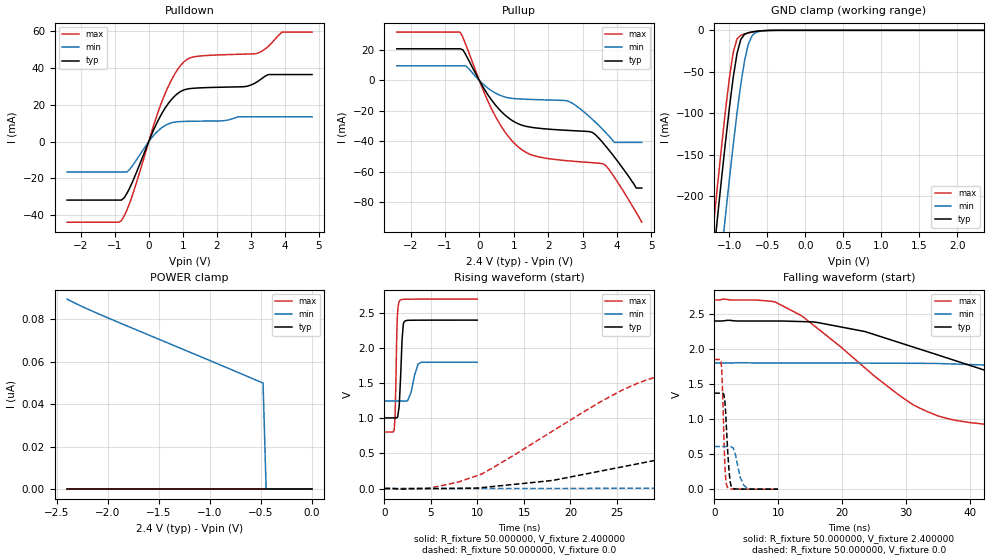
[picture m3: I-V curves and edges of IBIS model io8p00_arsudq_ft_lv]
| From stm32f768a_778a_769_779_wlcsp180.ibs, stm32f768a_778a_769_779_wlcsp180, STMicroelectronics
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|   Model io8p00_arsudq_ft_lv
[Model]  io8p00_arsudq_ft_lv
Model_type I/O
Polarity   Non-Inverting
Enable   Active-Low
Vinl =   0.720000V
Vinh =   1.680000V
Vmeas =  1.200000V
Cref =   50.000000pF
Rref =   100.000000M
Vref =   0.0V
C_comp   2.238800pF   2.178700pF   2.334000pF
[Temperature Range]   25.000000   0.125000k   -40.000000
[Pullup Reference]   2.400000V   1.800000V   2.700000V
[Pulldown Reference]   0.0V   0.0V   0.0V
[POWER Clamp Reference]   2.400000V   1.800000V   2.700000V
[GND Clamp Reference]   0.0V   0.0V   0.0V
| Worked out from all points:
|   slope of the pulldown table from 0 to 0.36 V, typ, clamps not added: 25 ohm
|   slope of the pullup table from 0 to 0.36 V, typ, clamps not added: 27.7 ohm
|   GND clamp passes 1 mA (typ) near -0.62 V on its own axis
|   rising waveform, R_fixture 50.000000, V_fixture 2.400000: 20-80 % time 271ps typ, 604ps min, 183ps max; typ from 1.01 V to 2.4 V
|   rising waveform, R_fixture 50.000000, V_fixture 0.0: 20-80 % time 32.8ns typ, 82.1ns min, 14.3ns max; typ from 0 V to 1.37 V
|   falling waveform, R_fixture 50.000000, V_fixture 2.400000: 20-80 % time 29.4ns typ, 74.3ns min, 15.7ns max; typ from 2.4 V to 1.01 V
|   falling waveform, R_fixture 50.000000, V_fixture 0.0: 20-80 % time 523ps typ, 976ps min, 385ps max; typ from 1.37 V to 0 V
[Pulldown]
|Voltage   I(typ)   I(min)   I(max)
-2.4V     -31.73mA   -16.51mA   -43.74mA
-800mV    -31.73mA   -16.51mA   -42.87mA
-480mV    -21.98mA   -13.17mA   -29.21mA
80mV      3.63mA     1.966mA    5.014mA
480mV     18.16mA    8.738mA    26.02mA
800mV     25.38mA    10.72mA    37.77mA
1.12V     28.53mA    11.02mA    44.6mA
2.8V      29.84mA    13.49mA    47.53mA
3.2V      32.65mA    13.49mA    48.05mA
3.52V     36.43mA    13.49mA    51.84mA
3.92V     36.43mA    13.49mA    59.49mA
4.8V      36.43mA    13.49mA    59.49mA
[Pullup]
|Voltage   I(typ)   I(min)   I(max)
-2.4V     20.89mA    9.66mA     31.9mA
-560mV    20.89mA    9.66mA     31.9mA
-400mV    17.28mA    9.66mA     24.07mA
320mV     -11.75mA   -6.207mA   -17.08mA
960mV     -26.47mA   -11.82mA   -40.02mA
1.52V     -30.88mA   -12.51mA   -49.05mA
2.56V     -32.88mA   -13.48mA   -52.9mA
3.28V     -34.19mA   -25.52mA   -54.18mA
3.6V      -41.31mA   -32.62mA   -54.97mA
3.92V     -50.33mA   -40.8mA    -63.62mA
4.56V     -70.9mA    -40.8mA    -87.08mA
4.72V     -70.9mA    -40.8mA    -93.4mA
[GND_clamp]
|Voltage   I(typ)   I(min)   I(max)
-2.4V     -1.424A    -1.508A    -1.393A
-1.25V    -311.2mA   -401.9mA   -273.3mA
-1.2V     -265.4mA   -356.1mA   -227.2mA
-1.15V    -220.4mA   -310.8mA   -181.9mA
-1.1V     -176.3mA   -266.2mA   -137.9mA
-1.05V    -133.8mA   -222.5mA   -95.87mA
-950mV    -57.3mA    -138.9mA   -26.98mA
-900mV    -28.27mA   -100.4mA   -10.59mA
-850mV    -11.01mA   -65.54mA   -5.958mA
-750mV    -2.834mA   -16.5mA    -3.178mA
-600mV    -750uA     -1.164mA   -738.3uA
2.35V     0A         0A         0A
[POWER_clamp]
|Voltage   I(typ)   I(min)   I(max)
-2.4V     0A         89.62nA    0A
-2.04V    0A         81.57nA    0A
-480mV    0A         50.01nA    0A
-450mV    0A         0A         0A
0V        0A         0A         0A
[Ramp]
| variable   typ   min   max
dV/dt_r  0.82248/32.81014n   0.36278/85.09684n   1.11120/14.28647n
dV/dt_f  0.83724/29.41275n   0.32736/79.44038n   1.13725/15.71354n
R_load = 50.000000
[Rising Waveform]
R_fixture= 50.000000
V_fixture= 2.400000
V_fixture_min= 1.800000
V_fixture_max= 2.700000
|time   V(typ)   V(min)   V(max)
0s        1.006V     1.247V     804.6mV
1.041ns   1.006V     1.247V     831.5mV
1.141ns   1.006V     1.247V     1.042V
1.381ns   1.014V     1.247V     2.44V
1.642ns   1.336V     1.247V     2.678V
1.902ns   2.139V     1.247V     2.694V
2.162ns   2.384V     1.245V     2.696V
2.843ns   2.398V     1.367V     2.698V
3.664ns   2.399V     1.778V     2.699V
9.97ns    2.4V       1.8V       2.7V
[Rising Waveform]
R_fixture= 50.000000
V_fixture= 0.0
V_fixture_min= 0.0
V_fixture_max= 0.0
|time   V(typ)   V(min)   V(max)
0s        4.248nV    257.3nV    1.628nV
4.505ns   -217.8uV   6.586uV    1.418mV
10.01ns   6.2mV      -65.69uV   185.4mV
26.53ns   333.6mV    3.98mV     1.461V
31.53ns   465.2mV    8.867mV    1.657V
36.54ns   613.4mV    23.12mV    1.741V
58.06ns   1.116V     86.41mV    1.832V
77.08ns   1.308V     179.6mV    1.847V
148.1ns   1.368V     490.1mV    1.852V
249.2ns   1.37V      609.1mV    1.852V
[Falling Waveform]
R_fixture= 50.000000
V_fixture= 2.400000
V_fixture_min= 1.800000
V_fixture_max= 2.700000
|time   V(typ)   V(min)   V(max)
0s        2.4V       1.8V       2.7V
9.51ns    2.4V       1.8V       2.672V
16.02ns   2.381V     1.8V       2.305V
31.03ns   2.03V      1.796V     1.208V
36.54ns   1.868V     1.789V     1.006V
43.54ns   1.66V      1.769V     914.2mV
59.56ns   1.248V     1.713V     849.5mV
88.09ns   1.07V      1.555V     816.7mV
124.1ns   1.025V     1.384V     807.4mV
249.2ns   1.006V     1.247V     804.6mV
[Falling Waveform]
R_fixture= 50.000000
V_fixture= 0.0
V_fixture_min= 0.0
V_fixture_max= 0.0
|time   V(typ)   V(min)   V(max)
0s        1.37V      609.1mV    1.852V
1.061ns   1.37V      609.1mV    1.82V
1.241ns   1.37V      609mV      1.572V
1.682ns   1.234V     608.8mV    323.1mV
1.842ns   1.005V     608.5mV    114.2mV
2.062ns   623mV      608.4mV    30.59mV
2.482ns   118.9mV    610.7mV    4.402mV
2.843ns   18.05mV    594.2mV    1.776mV
4.645ns   492.8uV    52.86mV    416.3uV
9.97ns    4.248nV    257.3nV    1.628nV
